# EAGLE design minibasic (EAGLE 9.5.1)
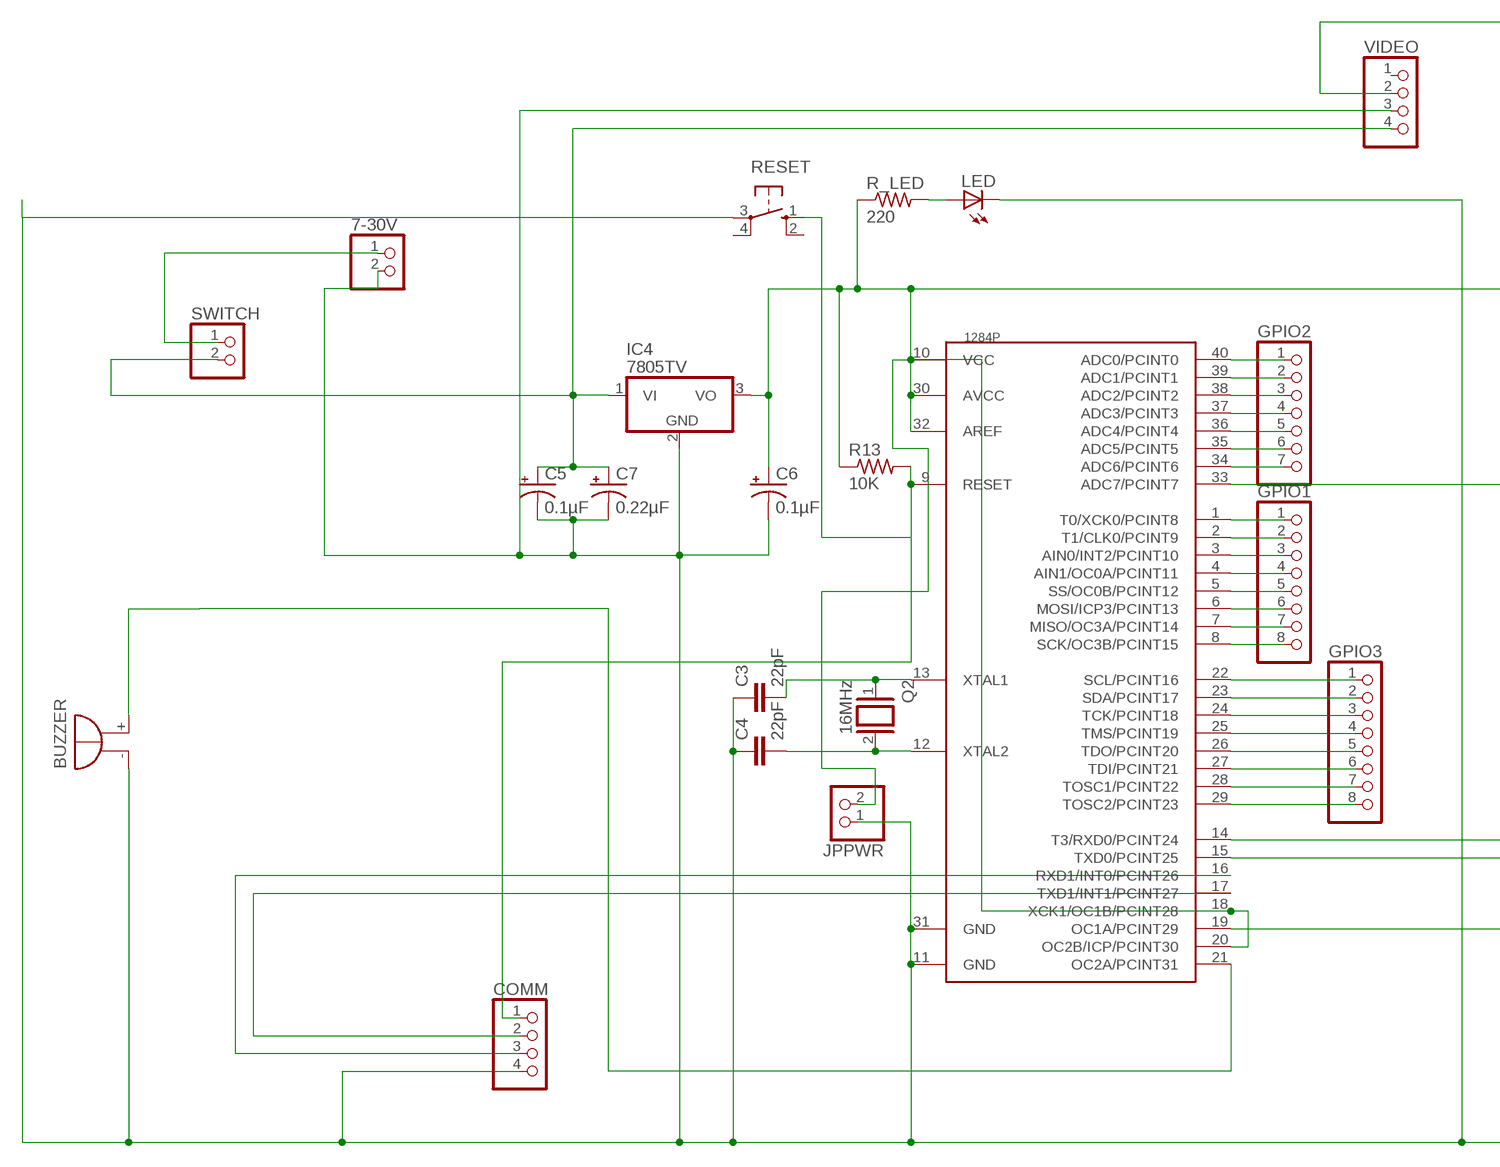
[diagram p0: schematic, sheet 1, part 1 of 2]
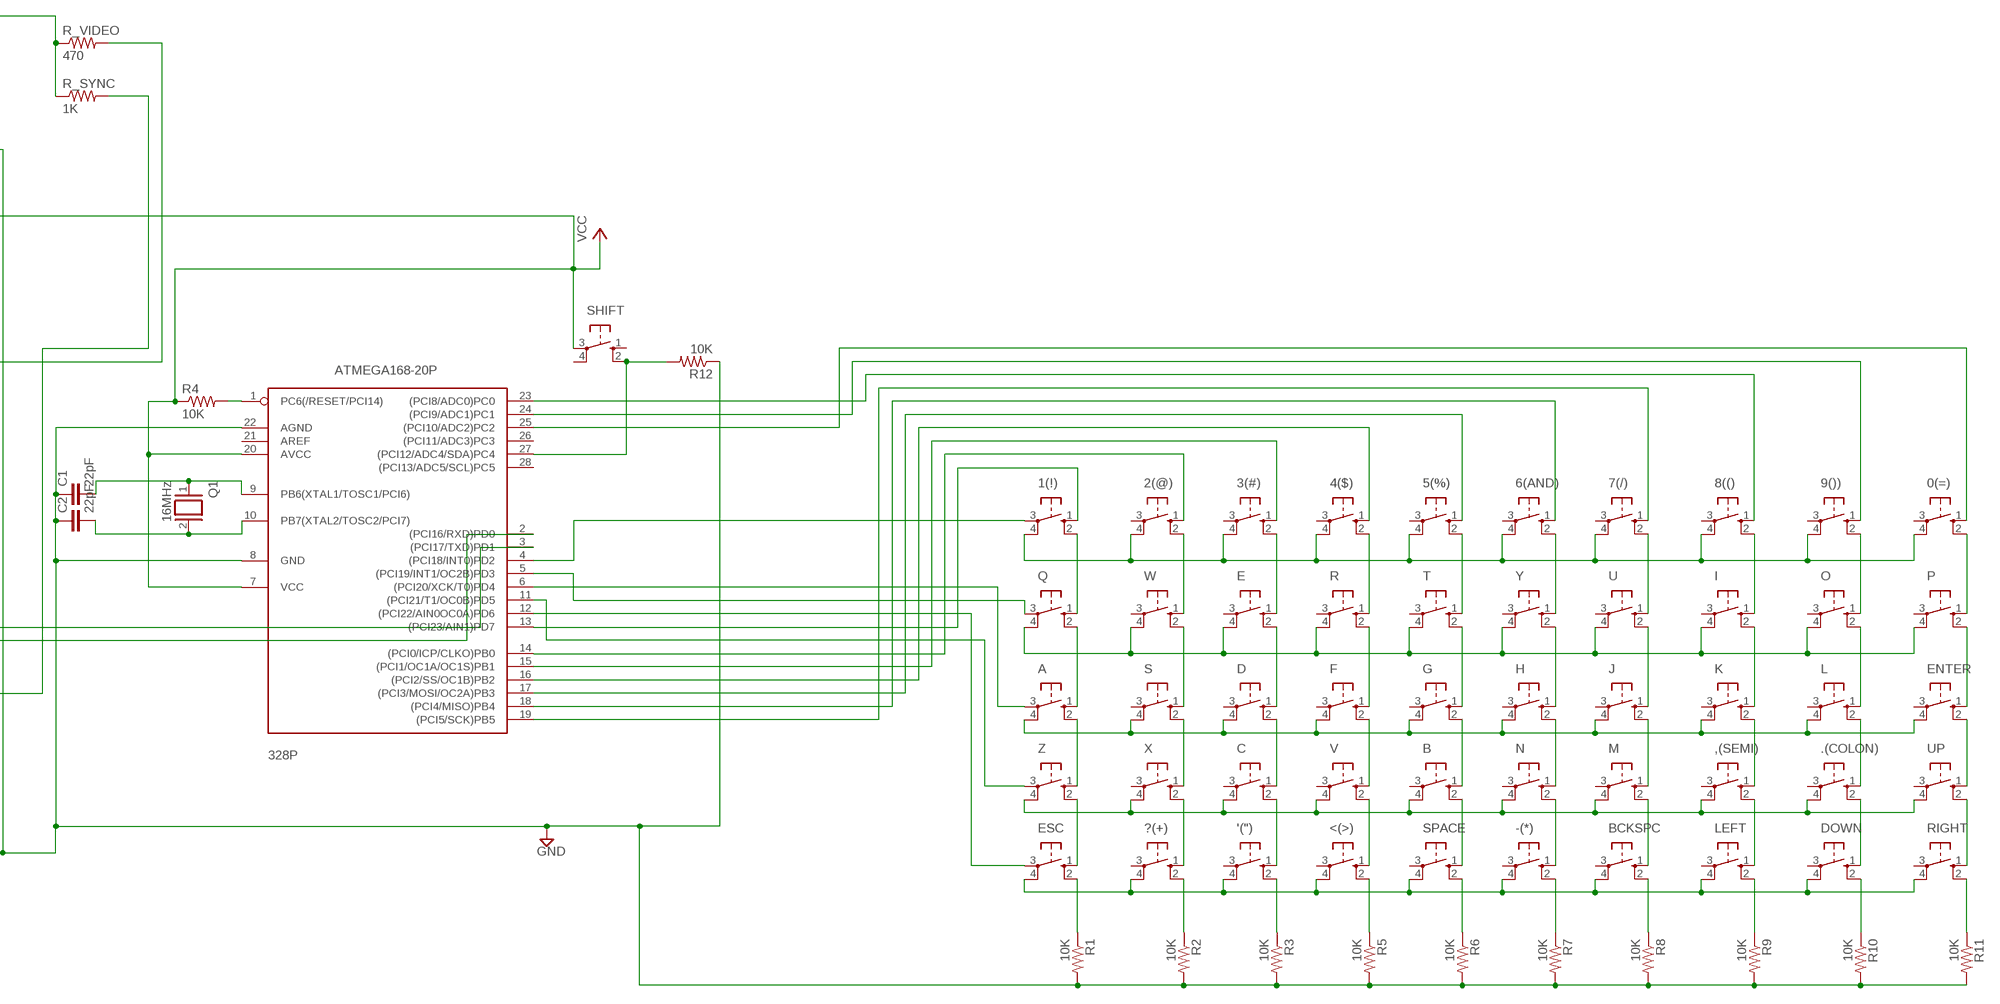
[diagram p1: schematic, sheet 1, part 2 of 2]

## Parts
0(=)  10-XX  [B3F-10XX]
1(!)  10-XX  [B3F-10XX]
2(@)  10-XX  [B3F-10XX]
3(#)  10-XX  [B3F-10XX]
4($)  10-XX  [B3F-10XX]
5(%)  10-XX  [B3F-10XX]
6(AND)  10-XX  [B3F-10XX]
7(/)  10-XX  [B3F-10XX]
7-30V  PINHD-1X2  [1X02]
8(()  10-XX  [B3F-10XX]
9())  10-XX  [B3F-10XX]
328P  ATMEGA168-20P  [DIL28-3]
1284P  MEGA1284P  [DIL40]
'(")  10-XX  [B3F-10XX]
,(SEMI)  10-XX  [B3F-10XX]
-(*)  10-XX  [B3F-10XX]
.(COLON)  10-XX  [B3F-10XX]
<(>)  10-XX  [B3F-10XX]
?(+)  10-XX  [B3F-10XX]
A  10-XX  [B3F-10XX]
B  10-XX  [B3F-10XX]
BCKSPC  10-XX  [B3F-10XX]
BUZZER  F/QMBIII  [F/QMBIII]
C  10-XX  [B3F-10XX]
C1  22pF  C-EU050-050X075  [C050-050X075]
C2  22pF  C-EU050-050X075  [C050-050X075]
C3  22pF  C-EU050-050X075  [C050-050X075]
C4  22pF  C-EU050-050X075  [C050-050X075]
C5  0.1µF  CPOL-USE2-4  [E2-4]
C6  0.1µF  CPOL-USE2-4  [E2-4]
C7  0.22µF  CPOL-USE2.5-5  [E2,5-5]
COMM  PINHD-1X4  [1X04]
D  10-XX  [B3F-10XX]
DOWN  10-XX  [B3F-10XX]
E  10-XX  [B3F-10XX]
ENTER  10-XX  [B3F-10XX]
ESC  10-XX  [B3F-10XX]
F  10-XX  [B3F-10XX]
G  10-XX  [B3F-10XX]
GPIO1  PINHD-1X8  [1X08]
GPIO2  PINHD-1X7  [1X07]
GPIO3  PINHD-1X8  [1X08]
H  10-XX  [B3F-10XX]
I  10-XX  [B3F-10XX]
IC4  7805TV  [TO220V]
J  10-XX  [B3F-10XX]
JPPWR  PINHD-1X2  [1X02]
K  10-XX  [B3F-10XX]
L  10-XX  [B3F-10XX]
LED  LED3MM  [LED3MM]
LEFT  10-XX  [B3F-10XX]
M  10-XX  [B3F-10XX]
N  10-XX  [B3F-10XX]
O  10-XX  [B3F-10XX]
P  10-XX  [B3F-10XX]
Q  10-XX  [B3F-10XX]
Q1  16MHz  XTAL/S  [QS]
Q2  16MHz  XTAL/S  [QS]
R  10-XX  [B3F-10XX]
R1  10K  R-US_0207/10  [0207/10]
R2  10K  R-US_0207/10  [0207/10]
R3  10K  R-US_0207/10  [0207/10]
R4  10K  R-US_0207/10  [0207/10]
R5  10K  R-US_0207/10  [0207/10]
R6  10K  R-US_0207/10  [0207/10]
R7  10K  R-US_0207/10  [0207/10]
R8  10K  R-US_0207/10  [0207/10]
R9  10K  R-US_0207/10  [0207/10]
R10  10K  R-US_0207/10  [0207/10]
R11  10K  R-US_0207/10  [0207/10]
R12  10K  R-US_0207/10  [0207/10]
R13  10K  R-US_0207/10  [0207/10]
R_LED  220  R-US_0207/10  [0207/10]
R_SYNC  1K  R-US_0207/10  [0207/10]
R_VIDEO  470  R-US_0207/10  [0207/10]
RESET  10-XX  [B3F-10XX]
RIGHT  10-XX  [B3F-10XX]
S  10-XX  [B3F-10XX]
SHIFT  10-XX  [B3F-10XX]
SPACE  10-XX  [B3F-10XX]
SWITCH  PINHD-1X2  [1X02]
T  10-XX  [B3F-10XX]
U  10-XX  [B3F-10XX]
UP  10-XX  [B3F-10XX]
V  10-XX  [B3F-10XX]
VIDEO  PINHD-1X4  [1X04]
W  10-XX  [B3F-10XX]
X  10-XX  [B3F-10XX]
Y  10-XX  [B3F-10XX]
Z  10-XX  [B3F-10XX]

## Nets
GND: 7-30V.2 328P.8(GND) 328P.22(AGND) 1284P.11(GND) 1284P.31(GND) BUZZER.-(+) C1.1 C2.1 C3.1 C4.1 C5.- C6.- C7.- COMM.4 IC4.2(GND) JPPWR.1 LED.K(C) R1.2 R2.2 R3.2 R5.2 R6.2 R7.2 R8.2 R9.2 R10.2 R11.2 R12.1 RESET.3(P) VIDEO.3
N$1: 1(!).2(S1) Q.1(S)
N$2: A.1(S) Q.2(S1)
N$3: A.2(S1) Z.1(S)
N$4: ESC.1(S) Z.2(S1)
N$5: 328P.1(PC6(/RESET/PCI14)) R4.2
N$6: ?(+).1(S) X.2(S1)
N$7: S.2(S1) X.1(S)
N$8: 328P.9(PB6(XTAL1/TOSC1/PCI6)) C1.2 Q1.1
N$9: 328P.10(PB7(XTAL2/TOSC2/PCI7)) C2.2 Q1.2
N$10: S.1(S) W.2(S1)
N$11: 2(@).2(S1) W.1(S)
N$12: '(").1(S) C.2(S1)
N$13: C.1(S) D.2(S1)
N$14: D.1(S) E.2(S1)
N$15: 3(#).2(S1) E.1(S)
N$16: 4($).2(S1) R.1(S)
N$17: F.1(S) R.2(S1)
N$18: F.2(S1) V.1(S)
N$19: <(>).1(S) V.2(S1)
N$20: B.2(S1) SPACE.1(S)
N$21: B.1(S) G.2(S1)
N$22: G.1(S) T.2(S1)
N$23: 5(%).2(S1) T.1(S)
N$24: 6(AND).2(S1) Y.1(S)
N$25: H.1(S) Y.2(S1)
N$26: H.2(S1) N.1(S)
N$27: -(*).1(S) N.2(S1)
N$28: BCKSPC.1(S) M.2(S1)
N$29: J.2(S1) M.1(S)
N$30: J.1(S) U.2(S1)
N$31: 7(/).2(S1) U.1(S)
N$32: 8(().2(S1) I.1(S)
N$33: I.2(S1) K.1(S)
N$34: ,(SEMI).1(S) K.2(S1)
N$35: ,(SEMI).2(S1) LEFT.1(S)
N$36: .(COLON).2(S1) DOWN.1(S)
N$37: .(COLON).1(S) L.2(S1)
N$38: L.1(S) O.2(S1)
N$39: 9()).2(S1) O.1(S)
N$40: 0(=).2(S1) P.1(S)
N$41: ENTER.1(S) P.2(S1)
N$42: ENTER.2(S1) UP.1(S)
N$43: RIGHT.1(S) UP.2(S1)
N$44: 0(=).4(P1) 1(!).4(P1) 2(@).4(P1) 3(#).4(P1) 4($).4(P1) 5(%).4(P1) 6(AND).4(P1) 7(/).4(P1) 8(().4(P1) 9()).4(P1)
N$45: 1(!).1(S) 328P.13((PCI23/AIN1)PD7)
N$46: E.4(P1) I.4(P1) O.4(P1) P.4(P1) Q.4(P1) R.4(P1) T.4(P1) U.4(P1) W.4(P1) Y.4(P1)
N$47: A.4(P1) D.4(P1) ENTER.4(P1) F.4(P1) G.4(P1) H.4(P1) J.4(P1) K.4(P1) L.4(P1) S.4(P1)
N$48: ,(SEMI).4(P1) .(COLON).4(P1) B.4(P1) C.4(P1) M.4(P1) N.4(P1) UP.4(P1) V.4(P1) X.4(P1) Z.4(P1)
N$49: '(").4(P1) -(*).4(P1) <(>).4(P1) ?(+).4(P1) BCKSPC.4(P1) DOWN.4(P1) ESC.4(P1) LEFT.4(P1) RIGHT.4(P1) SPACE.4(P1)
N$50: R11.1 RIGHT.2(S1)
N$51: DOWN.2(S1) R10.1
N$52: LEFT.2(S1) R9.1
N$53: BCKSPC.2(S1) R8.1
N$54: -(*).2(S1) R7.1
N$55: R6.1 SPACE.2(S1)
N$56: <(>).2(S1) R5.1
N$57: '(").2(S1) R3.1
N$58: ?(+).2(S1) R2.1
N$59: ESC.2(S1) R1.1
N$60: 2(@).1(S) 328P.14((PCI0/ICP/CLKO)PB0)
N$61: 1(!).3(P) 328P.4((PCI18/INT0)PD2)
N$62: 328P.5((PCI19/INT1/OC2B)PD3) Q.3(P)
N$63: 328P.6((PCI20/XCK/T0)PD4) A.3(P)
N$64: 328P.11((PCI21/T1/OC0B)PD5) Z.3(P)
N$65: 328P.12((PCI22/AIN0OC0A)PD6) ESC.3(P)
N$66: 5(%).1(S) 328P.17((PCI3/MOSI/OC2A)PB3)
N$67: 3(#).1(S) 328P.15((PCI1/OC1A/OC1S)PB1)
N$68: 4($).1(S) 328P.16((PCI2/SS/OC1B)PB2)
N$69: 6(AND).1(S) 328P.18((PCI4/MISO)PB4)
N$70: 7(/).1(S) 328P.19((PCI5/SCK)PB5)
N$71: 8(().1(S) 328P.23((PCI8/ADC0)PC0)
N$72: 9()).1(S) 328P.24((PCI9/ADC1)PC1)
N$73: 0(=).1(S) 328P.25((PCI10/ADC2)PC2)
N$74: 328P.27((PCI12/ADC4/SDA)PC4) R12.2 SHIFT.2(S1)
N$75: R_SYNC.1 R_VIDEO.1 VIDEO.2
N$76: C5.+ C7.+ IC4.1(VI) SWITCH.2 VIDEO.4
N$77: LED.A R_LED.2
N$78: 1284P.12(XTAL2) C4.2 Q2.2
N$79: 1284P.33(ADC7/PCINT7) R_VIDEO.2
N$80: 1284P.13(XTAL1) C3.2 Q2.1
N$81: 1284P.19(OC1A/PCINT29) R_SYNC.2
N$82: 328P.3((PCI17/TXD)PD1) 1284P.14(T3/RXD0/PCINT24)
N$83: 328P.2((PCI16/RXD)PD0) 1284P.15(TXD0/PCINT25)
N$84: 1284P.9(RESET) COMM.1 R13.2 RESET.1(S)
N$85: 7-30V.1 SWITCH.1
N$86: 1284P.16(RXD1/INT0/PCINT26) COMM.3
N$87: 1284P.17(TXD1/INT1/PCINT27) COMM.2
N$88: 1284P.21(OC2A/PCINT31) BUZZER.+(-)
N$89: 1284P.1(T0/XCK0/PCINT8) GPIO1.1
N$90: 1284P.2(T1/CLK0/PCINT9) GPIO1.2
N$91: 1284P.3(AIN0/INT2/PCINT10) GPIO1.3
N$92: 1284P.4(AIN1/OC0A/PCINT11) GPIO1.4
N$93: 1284P.5(SS/OC0B/PCINT12) GPIO1.5
N$94: 1284P.6(MOSI/ICP3/PCINT13) GPIO1.6
N$95: 1284P.7(MISO/OC3A/PCINT14) GPIO1.7
N$96: 1284P.8(SCK/OC3B/PCINT15) GPIO1.8
N$97: 1284P.40(ADC0/PCINT0) GPIO2.1
N$98: 1284P.39(ADC1/PCINT1) GPIO2.2
N$99: 1284P.38(ADC2/PCINT2) GPIO2.3
N$100: 1284P.37(ADC3/PCINT3) GPIO2.4
N$101: 1284P.36(ADC4/PCINT4) GPIO2.5
N$102: 1284P.35(ADC5/PCINT5) GPIO2.6
N$103: 1284P.34(ADC6/PCINT6) GPIO2.7
N$104: 1284P.22(SCL/PCINT16) GPIO3.1
N$105: 1284P.23(SDA/PCINT17) GPIO3.2
N$106: 1284P.24(TCK/PCINT18) GPIO3.3
N$107: 1284P.25(TMS/PCINT19) GPIO3.4
N$108: 1284P.26(TDO/PCINT20) GPIO3.5
N$109: 1284P.27(TDI/PCINT21) GPIO3.6
N$110: 1284P.28(TOSC1/PCINT22) GPIO3.7
N$111: 1284P.29(TOSC2/PCINT23) GPIO3.8
VCC: 328P.7(VCC) 328P.20(AVCC) 1284P.10(VCC) 1284P.18(XCK1/OC1B/PCINT28) 1284P.20(OC2B/ICP/PCINT30) 1284P.30(AVCC) 1284P.32(AREF) C6.+ IC4.3(VO) JPPWR.2 R4.1 R13.1 R_LED.1 SHIFT.3(P)
Unconnected: 0(=).3(P) 2(@).3(P) 3(#).3(P) 4($).3(P) 5(%).3(P) 6(AND).3(P) 7(/).3(P) 8(().3(P) 9()).3(P) 328P.21(AREF) 328P.26((PCI11/ADC3)PC3) 328P.28((PCI13/ADC5/SCL)PC5) '(").3(P) ,(SEMI).3(P) -(*).3(P) .(COLON).3(P) <(>).3(P) ?(+).3(P) B.3(P) BCKSPC.3(P) C.3(P) D.3(P) DOWN.3(P) E.3(P) ENTER.3(P) F.3(P) G.3(P) H.3(P) I.3(P) J.3(P) K.3(P) L.3(P) LEFT.3(P) M.3(P) N.3(P) O.3(P) P.3(P) R.3(P) RESET.2(S1) RESET.4(P1) RIGHT.3(P) S.3(P) SHIFT.1(S) SHIFT.4(P1) SPACE.3(P) T.3(P) U.3(P) UP.3(P) V.3(P) VIDEO.1 W.3(P) X.3(P) Y.3(P)

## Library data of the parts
0(=) 1(!) 2(@) 3(#) 4($) 5(%) 6(AND) 7(/) 8(() 9()) '(") ,(SEMI) -(*) .(COLON) <(>) ?(+) A B BCKSPC C D DOWN E ENTER ESC F G H I J K L LEFT M N O P Q R RESET RIGHT S SHIFT SPACE T U UP V W X Y Z = switch-omron:10-XX: OMRON SWITCH; MPN: B3F-1000; OC_FARNELL: 176432; OC_NEWARK: 36M3542
7-30V JPPWR SWITCH = pinhead:PINHD-1X2: PIN HEADER
328P = adafruit:ATMEGA168*P: MICROCONTROLLER 16 kBytes FLASH 1 kBytes SRAM 512 Bytes EEPROM USART 8-channel 10 bit ADC
1284P = 1284p:MEGA1284P: Atmel ATmega1284P 8-bit AVR Microcontroller
BUZZER = buzzer:F/QMBIII: BUZZER; OC_FARNELL: unknown; OC_NEWARK: unknown
C1-C4 = rcl:C-EU: CAPACITOR, European symbol; SPICEPREFIX: C
C5-C7 = adafruit:CPOL-US: POLARIZED CAPACITOR, American symbol
COMM VIDEO = pinhead:PINHD-1X4: PIN HEADER
GPIO1 GPIO3 = pinhead:PINHD-1X8: PIN HEADER
GPIO2 = pinhead:PINHD-1X7: PIN HEADER
IC4 = linear:78*: Positive VOLTAGE REGULATOR Source: http://cache.national.com/ds/LM/LM78L05.pdf http://www.fairchildsemi.com/ds/LM/LM7805.pdf
LED = adafruit:LED: LED
Q1 Q2 = special:XTAL/S: CRYSTAL
R1-R13 R_LED R_SYNC R_VIDEO = adafruit:R-US_: RESISTOR, American symbol

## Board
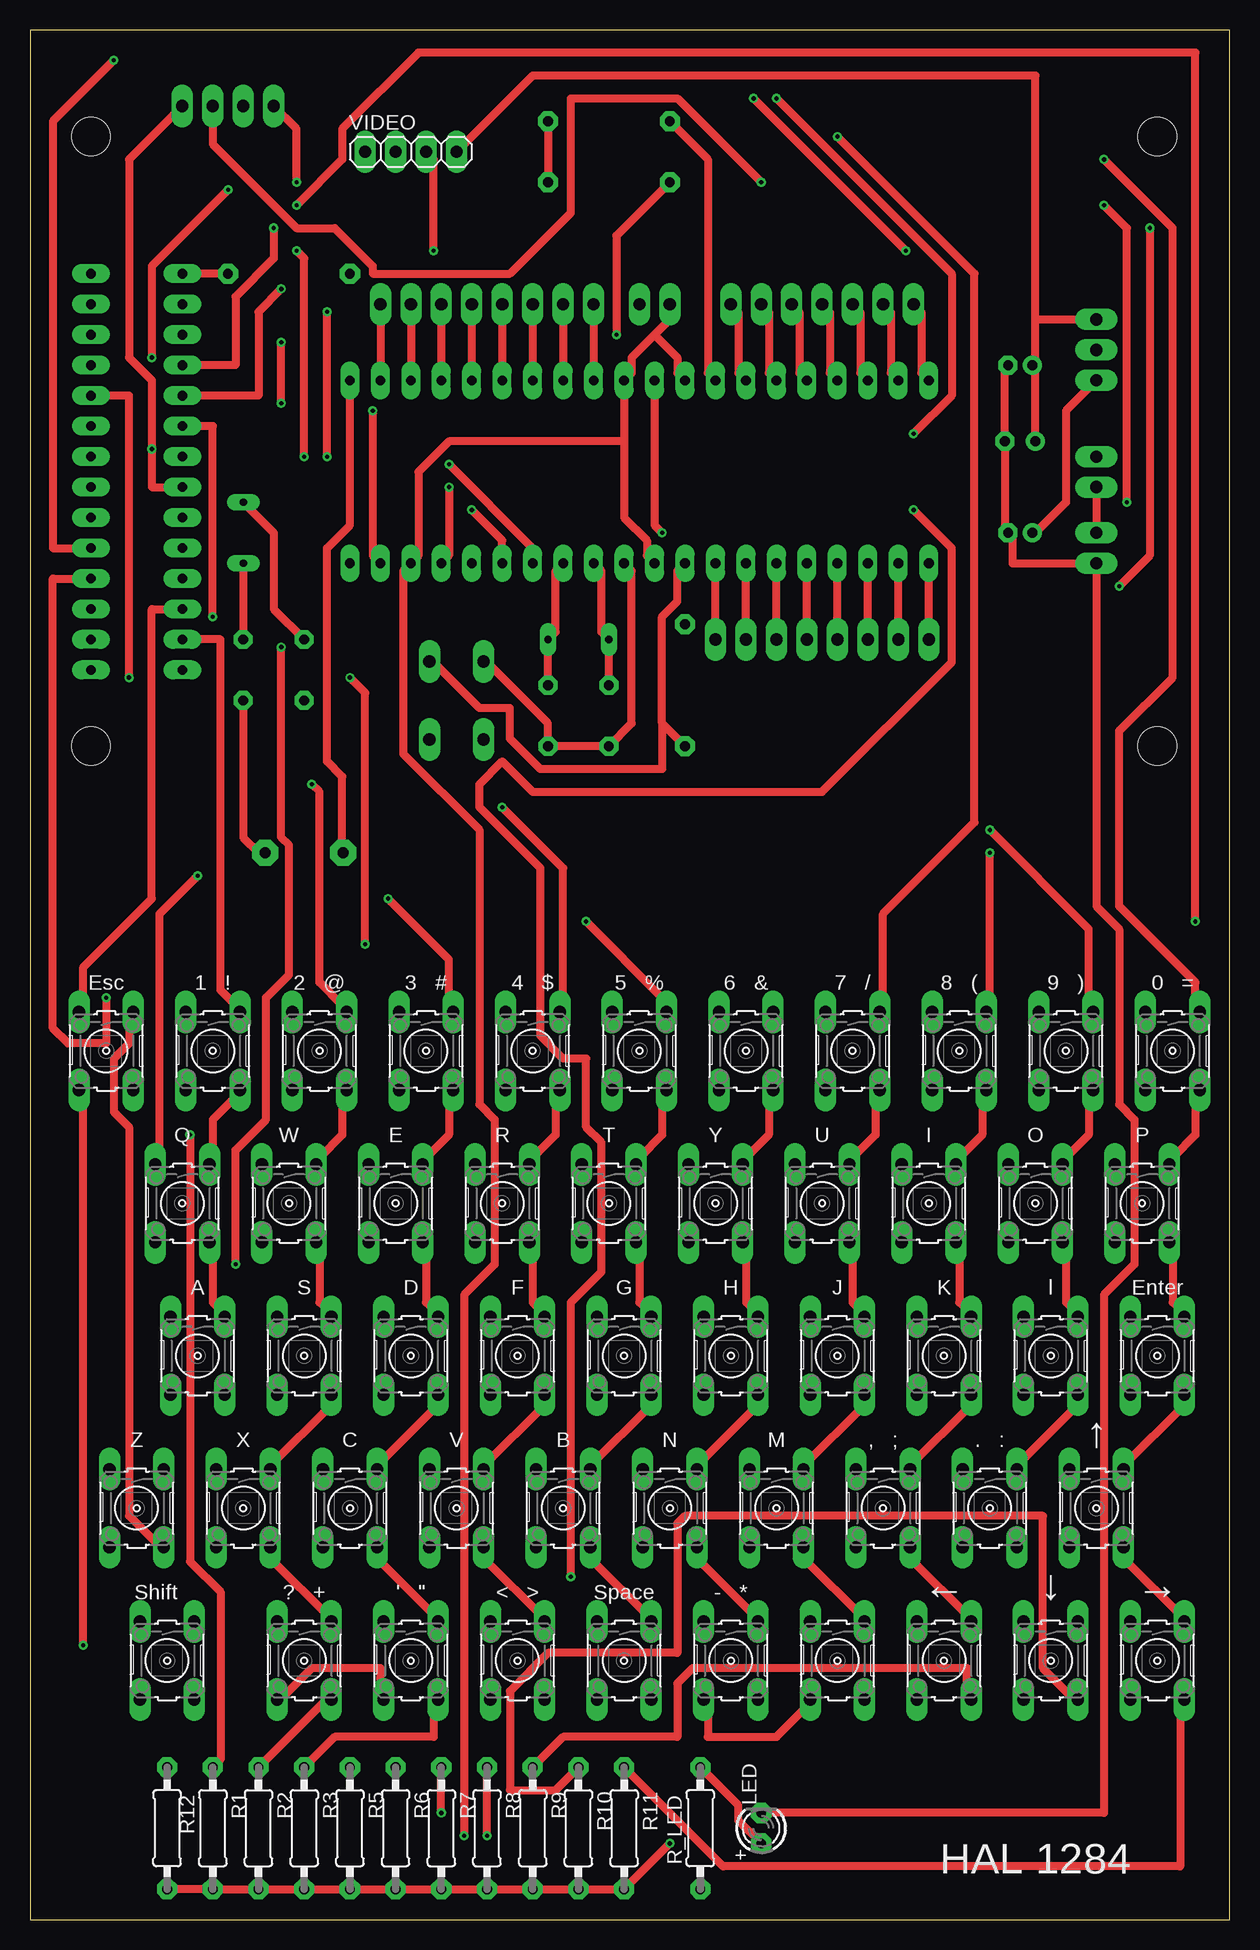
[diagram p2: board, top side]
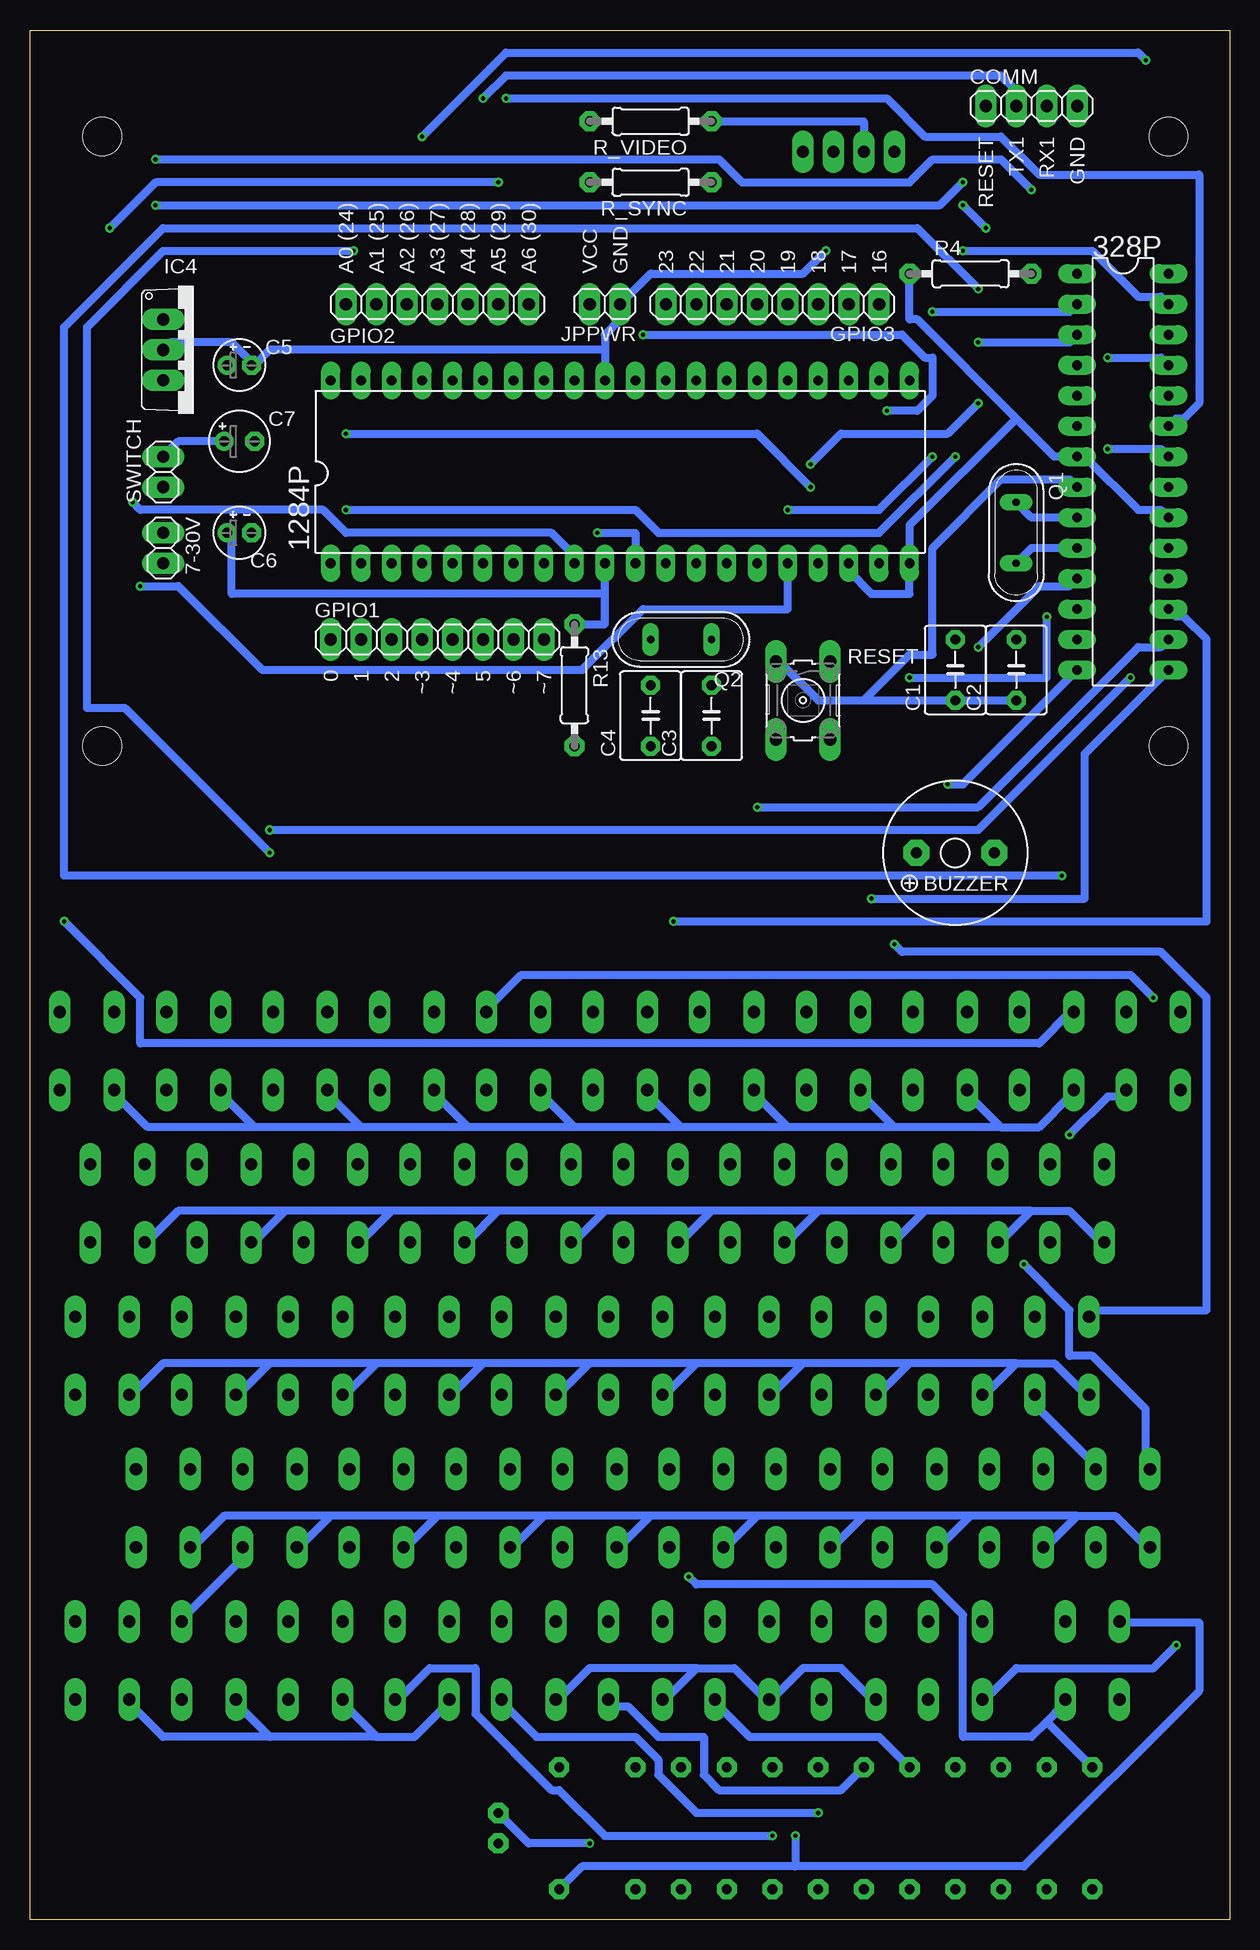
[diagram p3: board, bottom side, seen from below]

Size 100 x 157.47 mm. Coordinates in mm from the lower left corner, seen from the top.
Outline: 0,0 100,0 100,157.47 0,157.47 0,0
Copper layers (1*16): Top 0.035mm / dielectric 1.5mm / Bottom 0.035mm
Design rules "default *": minimum track width 26mil, minimum drill 0.35mm, track to track 26mil, track to pad 16mil, pad to pad 10mil, via to via 6mil, smd to smd 6mil, copper to edge 40mil, drill to drill 6mil, minimum pad ring 15mil, minimum via ring 8mil, stop-mask expansion 4mil, vias tented up to drill 0mil, thermal gap 10mil
Holes 3.2 mm at 5.08,148.59 93.98,148.59 5.08,97.79 93.98,97.79

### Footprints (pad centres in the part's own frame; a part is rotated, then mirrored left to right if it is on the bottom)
B3F-10XX = drill 1.016 long: 1 -3.251,2.261; 2 3.251,2.261; 3 -3.251,-2.261; 4 3.251,-2.261
1X02 = drill 1.016 long: 1 -1.27,0; 2 1.27,0
DIL28-3 = drill 0.813 long: 1 -16.51,-3.81; 2 -13.97,-3.81; 3 -11.43,-3.81; 4 -8.89,-3.81; 5 -6.35,-3.81; 6 -3.81,-3.81; 7 -1.27,-3.81; 8 1.27,-3.81; 9 3.81,-3.81; 10 6.35,-3.81; 11 8.89,-3.81; 12 11.43,-3.81; 13 13.97,-3.81; 14 16.51,-3.81; 15 16.51,3.81; 16 13.97,3.81; 17 11.43,3.81; 18 8.89,3.81; 19 6.35,3.81; 20 3.81,3.81; 21 1.27,3.81; 22 -1.27,3.81; 23 -3.81,3.81; 24 -6.35,3.81; 25 -8.89,3.81; 26 -11.43,3.81; 27 -13.97,3.81; 28 -16.51,3.81
DIL40 = drill 0.813 long: 1 -24.13,-7.62; 2 -21.59,-7.62; 3 -19.05,-7.62; 4 -16.51,-7.62; 5 -13.97,-7.62; 6 -11.43,-7.62; 7 -8.89,-7.62; 8 -6.35,-7.62; 9 -3.81,-7.62; 10 -1.27,-7.62; 11 1.27,-7.62; 12 3.81,-7.62; 13 6.35,-7.62; 14 8.89,-7.62; 15 11.43,-7.62; 16 13.97,-7.62; 17 16.51,-7.62; 18 19.05,-7.62; 19 21.59,-7.62; 20 24.13,-7.62; 21 24.13,7.62; 22 21.59,7.62; 23 19.05,7.62; 24 16.51,7.62; 25 13.97,7.62; 26 11.43,7.62; 27 8.89,7.62; 28 6.35,7.62; 29 3.81,7.62; 30 1.27,7.62; 31 -1.27,7.62; 32 -3.81,7.62; 33 -6.35,7.62; 34 -8.89,7.62; 35 -11.43,7.62; 36 -13.97,7.62; 37 -16.51,7.62; 38 -19.05,7.62; 39 -21.59,7.62; 40 -24.13,7.62
F/QMBIII = drill 0.914 pad 2.159 octagon: + 3.251,0; - -3.251,0
C050-050X075 = drill 0.813 octagon: 1 -2.54,0; 2 2.54,0
E2-4 = drill 0.813 pad 1.422: + -1.016,0 | drill 0.813 pad 1.422 octagon: - 1.016,0
E2,5-5 = drill 0.813 pad 1.6: + -1.27,0 | drill 0.813 pad 1.6 octagon: - 1.27,0
1X04 = drill 1.016 long: 1 -3.81,0; 2 -1.27,0; 3 1.27,0; 4 3.81,0
1X08 = drill 1.016 long: 1 -8.89,0; 2 -6.35,0; 3 -3.81,0; 4 -1.27,0; 5 1.27,0; 6 3.81,0; 7 6.35,0; 8 8.89,0
1X07 = drill 1.016 long: 1 -7.62,0; 2 -5.08,0; 3 -2.54,0; 4 0,0; 5 2.54,0; 6 5.08,0; 7 7.62,0
TO220V = drill 1.016 long: 1 -2.54,-2.54; 2 0,-2.54; 3 2.54,-2.54
LED3MM = drill 0.813 pad 1.676 octagon: A -1.27,0; K 1.27,0
QS = drill 0.61 long: 1 -2.54,0; 2 2.54,0
0207/10 = drill 0.813 pad 1.676 octagon: 1 -5.08,0; 2 5.08,0

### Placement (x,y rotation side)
0(=)  95.25,72.39 270 top
1(!)  15.24,72.39 270 top
2(@)  24.13,72.39 270 top
3(#)  33.02,72.39 270 top
4($)  41.91,72.39 270 top
5(%)  50.8,72.39 270 top
6(AND)  59.69,72.39 270 top
7(/)  68.58,72.39 270 top
7-30V  88.9,114.3 270 bottom
8(()  77.47,72.39 270 top
9())  86.36,72.39 270 top
328P  8.89,120.65 270 bottom
1284P  50.8,120.65 0 bottom
'(")  31.75,21.59 270 top
,(SEMI)  71.12,34.29 270 top
-(*)  58.42,21.59 270 top
.(COLON)  80.01,34.29 270 top
<(>)  40.64,21.59 270 top
?(+)  22.86,21.59 270 top
A  13.97,46.99 270 top
B  44.45,34.29 270 top
BCKSPC  67.31,21.59 270 top
BUZZER  22.86,88.9 180 bottom
C  26.67,34.29 270 top
C1  22.86,104.14 90 bottom
C2  17.78,104.14 90 bottom
C3  43.18,100.33 90 bottom
C4  48.26,100.33 90 bottom
C5  82.55,129.54 0 bottom
C6  82.55,115.57 0 bottom
C7  82.55,123.19 0 bottom
COMM  16.51,151.13 0 bottom
D  31.75,46.99 270 top
DOWN  85.09,21.59 270 top
E  30.48,59.69 270 top
ENTER  93.98,46.99 270 top
ESC  6.35,72.39 270 top
F  40.64,46.99 270 top
G  49.53,46.99 270 top
GPIO1  66.04,106.68 0 bottom
GPIO2  66.04,134.62 0 bottom
GPIO3  38.1,134.62 180 bottom
H  58.42,46.99 270 top
I  74.93,59.69 270 top
IC4  86.36,130.81 270 bottom
J  67.31,46.99 270 top
JPPWR  52.07,134.62 180 bottom
K  76.2,46.99 270 top
L  85.09,46.99 270 top
LED  60.96,7.62 90 top
LEFT  76.2,21.59 270 top
M  62.23,34.29 270 top
N  53.34,34.29 270 top
O  83.82,59.69 270 top
P  92.71,59.69 270 top
Q  12.7,59.69 270 top
Q1  17.78,115.57 270 bottom
Q2  45.72,106.68 180 bottom
R  39.37,59.69 270 top
R1  15.24,7.62 270 top
R2  19.05,7.62 270 top
R3  22.86,7.62 270 top
R4  21.59,137.16 0 bottom
R5  26.67,7.62 270 top
R6  30.48,7.62 270 top
R7  34.29,7.62 270 top
R8  38.1,7.62 270 top
R9  41.91,7.62 270 top
R10  45.72,7.62 270 top
R11  49.53,7.62 270 top
R12  11.43,7.62 90 top
R13  54.61,102.87 270 bottom
R_LED  55.88,7.62 90 top
R_SYNC  48.26,144.78 180 bottom
R_VIDEO  48.26,149.86 180 bottom
RESET  35.56,101.6 270 bottom
RIGHT  93.98,21.59 270 top
S  22.86,46.99 270 top
SHIFT  11.43,21.59 270 top
SPACE  49.53,21.59 270 top
SWITCH  88.9,120.65 90 bottom
T  48.26,59.69 270 top
U  66.04,59.69 270 top
UP  88.9,34.29 270 top
V  35.56,34.29 270 top
VIDEO  31.75,147.32 0 top
W  21.59,59.69 270 top
X  17.78,34.29 270 top
Y  57.15,59.69 270 top
Z  8.89,34.29 270 top

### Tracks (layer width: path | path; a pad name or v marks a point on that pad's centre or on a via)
GND  (via drill 0.35)
  Top 0.66: 328P.8 10.16,119.38 v10.16,122.56 10.16,128.27 8.25,130.18 8.25,146.69 COMM.4 | C2.1 17.78,90.17 19.05,88.9 BUZZER.- | 1284P.11 50.16,112.4 50.16,99.69 C4.1 C3.1 43.18,99.69 38.1,104.78 RESET.3 | R12.1 R1.2 R2.2 R3.2 R5.2 R6.2 R7.2 R8.2 R9.2 R10.2 R11.2 v53.34,6.35 | C5.- 81.28,129.54 C7.- 81.28,115.57 C6.- 81.91,115.57 81.91,113.03 7-30V.2 88.9,84.45 90.8,82.55 90.8,67.94 92.07,66.67 92.07,54.61 89.53,52.07 89.53,8.89 LED.K | VIDEO.3 33.66,146.69 v33.66,139.06 | v52.71,115.57 52.07,116.21 1284P.31
  Bottom 0.66: 328P.22 5.72,122.56 v10.16,122.56 | C2.1 C1.1 30.48,101.6 | 30.48,101.6 34.29,101.6 37.47,104.78 RESET.3 | 328P.8 13.33,120.01 19.05,120.01 24.76,114.3 24.76,105.41 26.67,105.41 30.48,101.6 | LED.K 58.42,6.35 v53.34,6.35 | IC4.2 88.27,131.44 83.19,131.44 81.28,129.54 | 52.07,130.81 52.07,132.08 50.8,133.35 JPPWR.1 48.26,137.16 35.56,137.16 v33.66,139.06 | 52.07,130.81 1284P.31 | 81.28,129.54 80.01,130.81 52.07,130.81 | 81.28,129.54 C5.- | 1284P.11 49.53,115.57 v52.71,115.57
N$1
  Top 0.66: Q.1 15.24,63.5 15.24,66.67 17.14,68.58 1(!).2
N$2
  Top 0.66: A.1 15.88,50.8 15.24,51.44 15.24,55.88 Q.2
N$3
  Bottom 0.66: Z.1 11.43,38.1 16.51,43.18 A.2
N$4
  Top 0.66: Z.2 10.79,31.12 8.25,33.66 8.25,66.04 6.99,67.31 6.99,71.75 8.25,73.03 8.25,75.56 ESC.1
N$5
  Top 0.66: R4.2 328P.1
N$6
  Top 0.66: ?(+).1 24.76,25.4 20.32,29.84 20.32,30.48 X.2
N$7
  Top 0.66: X.1 20.32,38.1 24.76,42.55 24.76,43.18 S.2
N$8
  Top 0.66: C1.2 20.32,109.22 20.32,115.57 Q1.1
  Bottom 0.66: Q1.1 16.51,116.84 328P.9
N$9
  Top 0.66: Q1.2 C2.2
  Bottom 0.66: Q1.2 16.51,114.3 328P.10
N$10
  Top 0.66: S.1 24.76,50.8 24.13,51.44 24.13,55.88 W.2
N$11
  Top 0.66: W.1 24.13,63.5 26.04,65.41 26.04,68.58 2(@).2
N$12
  Top 0.66: '(").1 33.66,25.4 29.21,29.84 29.21,30.48 C.2
N$13
  Top 0.66: C.1 29.21,38.1 33.66,42.55 33.66,43.18 D.2
N$14
  Top 0.66: D.1 33.66,50.8 33.02,51.44 33.02,55.88 E.2
N$15
  Top 0.66: E.1 33.02,63.5 34.93,65.41 34.93,68.58 3(#).2
N$16
  Top 0.66: R.1 41.91,63.5 43.82,65.41 43.82,68.58 4($).2
N$17
  Top 0.66: F.1 42.55,50.8 41.91,51.44 41.91,55.88 R.2
N$18
  Top 0.66: V.1 38.1,38.1 42.55,42.55 42.55,43.18 F.2
N$19
  Top 0.66: <(>).1 42.55,25.4 38.1,29.84 38.1,30.48 V.2
N$20
  Top 0.66: SPACE.1 51.44,25.4 46.99,29.84 46.99,30.48 B.2
N$21
  Top 0.66: B.1 46.99,38.1 51.44,42.55 51.44,43.18 G.2
N$22
  Top 0.66: G.1 51.44,50.8 50.8,51.44 50.8,55.88 T.2
N$23
  Top 0.66: T.1 50.8,63.5 52.71,65.41 52.71,68.58 5(%).2
N$24
  Top 0.66: Y.1 59.69,63.5 61.6,65.41 61.6,68.58 6(AND).2
N$25
  Top 0.66: H.1 60.32,50.8 59.69,51.44 59.69,55.88 Y.2
N$26
  Top 0.66: N.1 55.88,38.1 60.32,42.55 60.32,43.18 H.2
N$27
  Top 0.66: -(*).1 60.32,25.4 55.88,29.84 55.88,30.48 N.2
N$28
  Top 0.66: BCKSPC.1 69.21,25.4 64.77,29.84 64.77,30.48 M.2
N$29
  Top 0.66: M.1 64.77,38.1 69.21,42.55 69.21,43.18 J.2
N$30
  Top 0.66: J.1 69.21,50.8 68.58,51.44 68.58,55.88 U.2
N$31
  Top 0.66: U.1 68.58,63.5 70.48,65.41 70.48,68.58 7(/).2
N$32
  Top 0.66: I.1 77.47,63.5 79.38,65.41 79.38,68.58 8(().2
N$33
  Top 0.66: K.1 78.1,50.8 77.47,51.44 77.47,55.88 I.2
N$34
  Top 0.66: ,(SEMI).1 73.66,38.1 78.1,42.55 78.1,43.18 K.2
N$35
  Top 0.66: LEFT.1 78.1,25.4 73.66,29.84 73.66,30.48 ,(SEMI).2
N$36
  Bottom 0.66: DOWN.1 86.99,25.4 81.91,30.48 .(COLON).2
N$37
  Top 0.66: .(COLON).1 82.55,38.1 86.99,42.55 86.99,43.18 L.2
N$38
  Top 0.66: L.1 86.99,50.8 86.36,51.44 86.36,55.88 O.2
N$39
  Top 0.66: O.1 86.36,63.5 88.27,65.41 88.27,68.58 9()).2
N$40
  Top 0.66: P.1 95.25,63.5 97.16,65.41 97.16,68.58 0(=).2
N$41
  Top 0.66: ENTER.1 95.88,50.8 95.25,51.44 95.25,55.88 P.2
N$42
  Top 0.66: UP.1 91.44,38.1 95.88,42.55 95.88,43.18 ENTER.2
N$43
  Top 0.66: RIGHT.1 95.88,25.4 91.44,29.84 91.44,30.48 UP.2
N$44
  Bottom 0.66: 19.05,66.04 15.88,66.04 13.33,68.58 1(!).4 | 19.05,66.04 21.59,68.58 2(@).4 | 27.94,66.04 30.48,68.58 3(#).4 | 19.05,66.04 27.94,66.04 | 36.83,66.04 39.37,68.58 4($).4 | 27.94,66.04 36.83,66.04 | 45.72,66.04 48.26,68.58 5(%).4 | 36.83,66.04 45.72,66.04 | 54.61,66.04 57.15,68.58 6(AND).4 | 45.72,66.04 54.61,66.04 | 63.5,66.04 66.04,68.58 7(/).4 | 54.61,66.04 63.5,66.04 | 72.39,66.04 74.93,68.58 8(().4 | 63.5,66.04 72.39,66.04 | 81.28,66.04 83.82,68.58 9()).4 | 72.39,66.04 81.28,66.04 | 81.28,66.04 90.17,66.04 92.71,68.58 0(=).4
N$45
  Top 0.66: 328P.13 15.88,106.68 15.88,77.47 17.14,76.2 1(!).1
N$46
  Bottom 0.66: 16.51,59.05 13.33,59.05 10.79,56.52 Q.4 | 16.51,59.05 19.05,56.52 W.4 | 25.4,59.05 27.94,56.52 E.4 | 16.51,59.05 25.4,59.05 | 34.29,59.05 36.83,56.52 R.4 | 25.4,59.05 34.29,59.05 | 43.18,59.05 45.72,56.52 T.4 | 34.29,59.05 43.18,59.05 | 52.07,59.05 54.61,56.52 Y.4 | 43.18,59.05 52.07,59.05 | 60.96,59.05 63.5,56.52 U.4 | 52.07,59.05 60.96,59.05 | 69.85,59.05 72.39,56.52 I.4 | 60.96,59.05 69.85,59.05 | 78.74,59.05 81.28,56.52 O.4 | 69.85,59.05 78.74,59.05 | 78.74,59.05 87.63,59.05 90.17,56.52 P.4
N$47
  Bottom 0.66: 17.78,46.36 14.61,46.36 12.06,43.81 A.4 | 17.78,46.36 20.32,43.81 S.4 | 26.67,46.36 29.21,43.81 D.4 | 17.78,46.36 26.67,46.36 | 35.56,46.36 38.1,43.81 F.4 | 26.67,46.36 35.56,46.36 | 44.45,46.36 46.99,43.81 G.4 | 35.56,46.36 44.45,46.36 | 53.34,46.36 55.88,43.81 H.4 | 44.45,46.36 53.34,46.36 | 62.23,46.36 64.77,43.81 J.4 | 53.34,46.36 62.23,46.36 | 71.12,46.36 73.66,43.81 K.4 | 62.23,46.36 71.12,46.36 | 80.01,46.36 82.55,43.81 L.4 | 71.12,46.36 80.01,46.36 | 80.01,46.36 88.9,46.36 91.44,43.81 ENTER.4
N$48
  Bottom 0.66: 12.7,33.66 9.52,33.66 6.99,31.12 Z.4 | 12.7,33.66 15.24,31.12 X.4 | 21.59,33.66 24.13,31.12 C.4 | 12.7,33.66 21.59,33.66 | 30.48,33.66 33.02,31.12 V.4 | 21.59,33.66 30.48,33.66 | 39.37,33.66 41.91,31.12 B.4 | 30.48,33.66 39.37,33.66 | 48.26,33.66 50.8,31.12 N.4 | 39.37,33.66 48.26,33.66 | 57.15,33.66 59.69,31.12 M.4 | 48.26,33.66 57.15,33.66 | 66.04,33.66 68.58,31.12 ,(SEMI).4 | 57.15,33.66 66.04,33.66 | 74.93,33.66 77.47,31.12 .(COLON).4 | 66.04,33.66 74.93,33.66 | 74.93,33.66 83.82,33.66 86.36,31.12 UP.4
N$49  (via drill 0.35)
  Top 0.66: ?(+).4 20.95,18.41 23.49,20.95 29.21,20.95 29.21,18.41 '(").4 | v4.44,22.86 4.44,68.58 ESC.4 | BCKSPC.4 64.77,17.78 62.23,15.24 56.52,15.24 56.52,17.78 -(*).4
  Bottom 0.66: 71.12,15.24 67.94,15.24 65.41,17.78 BCKSPC.4 | 71.12,15.24 73.66,17.78 LEFT.4 | 80.01,15.24 82.55,17.78 DOWN.4 | 71.12,15.24 80.01,15.24 | 80.01,15.24 88.9,15.24 91.44,17.78 RIGHT.4 | 44.45,20.95 41.28,20.95 38.73,18.41 <(>).4 38.1,18.41 35.56,20.95 32.39,20.95 29.85,18.41 '(").4 | 44.45,20.95 46.99,18.41 SPACE.4 | 44.45,20.95 53.34,20.95 55.88,18.41 -(*).4 | v4.44,22.86 6.35,20.95 17.78,20.95 20.32,18.41 ?(+).4
N$50
  Top 0.66: R11.1 57.79,4.45 95.88,4.45 95.88,17.78 RIGHT.2
N$51
  Top 0.66: R10.1 43.82,10.79 40.01,10.79 40.01,19.05 43.18,22.23 53.98,22.23 53.98,33.02 54.61,33.66 84.45,33.66 84.45,20.95 86.99,18.41 DOWN.2
N$52
  Top 0.66: R9.1 44.45,15.24 53.98,15.24 53.98,19.69 55.25,20.95 78.1,20.95 78.1,18.41 LEFT.2
N$53  (via drill 0.35)
  Top 0.66: v38.1,6.98 R8.1
  Bottom 0.66: v38.1,6.98 52.07,6.98 55.88,10.79 56.52,10.79 62.87,17.14 62.87,20.95 66.67,20.95 69.21,18.41 BCKSPC.2
N$54  (via drill 0.35)
  Top 0.66: v34.29,8.89 R7.1
  Bottom 0.66: v34.29,8.89 44.45,8.89 47.62,12.06 47.62,13.33 49.53,15.24 57.79,15.24 60.32,17.78 -(*).2
N$55
  Bottom 0.66: R6.1 32.39,10.79 42.55,10.79 43.82,12.06 43.82,15.24 47.62,15.24 50.16,17.78 51.44,17.78 SPACE.2
N$56
  Bottom 0.66: R5.1 29.21,15.24 40.01,15.24 42.55,17.78 <(>).2
N$57
  Top 0.66: R3.1 25.4,15.24 33.66,15.24 33.66,17.78 '(").2
N$58
  Top 0.66: R2.1 24.76,18.41 ?(+).2
N$59  (via drill 0.35)
  Top 0.66: R1.1 15.88,13.33 15.88,27.3 13.33,29.84 v13.33,65.41
  Bottom 0.66: v13.33,65.41 10.16,68.58 8.89,68.58 ESC.2
N$60  (via drill 0.35)
  Top 0.66: v23.49,94.61 24.13,93.98 24.13,78.11 26.04,76.2 2(@).1
  Bottom 0.66: 328P.14 22.22,94.61 v23.49,94.61
N$61  (via drill 0.35)
  Top 0.66: 328P.4 17.14,129.54 17.14,135.25 20.32,138.43 v20.32,140.97 | v22.22,142.88 26.04,146.69 26.04,149.22 32.39,155.57 97.16,155.57 v97.16,83.19
  Bottom 0.66: v22.22,142.88 v20.32,140.97 | v97.16,83.19 90.8,76.83 90.8,73.03 15.88,73.03 13.33,75.56 1(!).3
N$62  (via drill 0.35)
  Top 0.66: 328P.5 19.05,127 19.05,133.98 v20.95,135.89 | v13.97,87 10.79,83.82 10.79,63.5 Q.3
  Bottom 0.66: v20.95,135.89 26.04,140.97 88.9,140.97 97.16,132.72 97.16,87 v13.97,87
N$63  (via drill 0.35)
  Top 0.66: 328P.6 15.24,124.46 v15.24,108.58 | v26.67,103.5 27.94,102.23 v27.94,81.28
  Bottom 0.66: v15.24,108.58 15.24,103.5 v26.67,103.5 | v27.94,81.28 27.3,80.64 5.72,80.64 1.91,76.83 1.91,50.8 11.43,50.8 A.3
N$64  (via drill 0.35)
  Top 0.66: v20.95,106.05 20.95,90.17 21.59,89.53 21.59,78.74 19.68,76.83 19.68,66.67 17.14,64.14 v17.14,54.61
  Bottom 0.66: 328P.11 13.33,111.12 15.88,111.12 v20.95,106.05 | v17.14,54.61 13.33,50.8 13.33,46.99 11.43,46.99 6.99,42.55 6.99,38.1 Z.3
N$65
  Top 0.66: 328P.12 10.16,109.22 10.16,85.09 4.44,79.38 4.44,76.2 ESC.3
N$66  (via drill 0.35)
  Top 0.66: v46.36,83.19 52.71,76.83 52.71,76.2 5(%).1
  Bottom 0.66: 328P.17 4.44,108.58 3.81,108.58 1.91,106.68 1.91,83.19 v46.36,83.19
N$67  (via drill 0.35)
  Top 0.66: v29.85,85.09 34.93,80.01 34.93,76.2 3(#).1
  Bottom 0.66: 328P.15 12.06,97.16 12.06,85.09 v29.85,85.09
N$68  (via drill 0.35)
  Top 0.66: v39.37,92.71 44.45,87.63 44.45,76.2 4($).1
  Bottom 0.66: 328P.16 5.72,106.05 7.62,106.05 20.95,92.71 v39.37,92.71
N$69  (via drill 0.35)
  Top 0.66: 328P.18 1.91,111.76 1.91,74.3 3.17,73.03 6.35,73.03 v6.35,76.83
  Bottom 0.66: v6.35,76.83 8.25,78.74 59.05,78.74 61.6,76.2 6(AND).1
N$70  (via drill 0.35)
  Top 0.66: 328P.19 1.91,114.3 1.91,149.86 v6.99,154.94 | v67.31,148.59 78.74,137.16 78.74,91.44 71.12,83.82 71.12,76.2 7(/).1
  Bottom 0.66: v6.99,154.94 7.62,155.57 60.32,155.57 v67.31,148.59
N$71  (via drill 0.35)
  Top 0.66: v73.02,139.06 v60.32,151.76 | v80.01,88.9 80.01,76.2 8(().1
  Bottom 0.66: 328P.23 4.44,125.09 3.81,125.09 2.54,126.37 2.54,145.41 15.88,145.41 19.05,148.59 25.4,148.59 28.57,151.76 v60.32,151.76 | v73.02,139.06 88.9,139.06 95.25,132.72 95.25,100.97 92.07,100.97 v80.01,88.9
N$72  (via drill 0.35)
  Top 0.66: 328P.24 8.25,127 v8.25,103.5 | v80.01,90.8 88.27,82.55 88.27,76.2 9()).1
  Bottom 0.66: v8.25,103.5 20.95,90.8 v80.01,90.8
N$73  (via drill 0.35)
  Top 0.66: v10.16,130.18 10.16,137.79 v16.51,144.15 | v89.53,146.69 95.25,140.97 95.25,103.5 90.8,99.06 90.8,84.45 97.16,78.11 97.16,76.2 0(=).1
  Bottom 0.66: 328P.25 5.72,130.18 v10.16,130.18 | v16.51,144.15 19.05,146.69 24.76,146.69 26.67,144.78 40.64,144.78 42.55,146.69 v89.53,146.69
N$74  (via drill 0.35)
  Top 0.66: v22.22,139.06 22.86,138.43 v22.86,121.92 | v73.66,117.47 76.83,114.3 76.83,104.78 66.04,93.98 41.91,93.98 39.37,96.52 37.47,94.61 37.47,92.71 42.55,87.63 42.55,73.66 44.45,71.75 46.36,71.75 46.36,66.04 47.62,64.77 47.62,53.97 45.09,51.44 v45.09,28.57
  Bottom 0.66: 328P.27 5.72,135.25 7.62,135.25 11.43,139.06 v22.22,139.06 | v22.86,121.92 29.21,115.57 47.62,115.57 49.53,117.47 v73.66,117.47 | v45.09,28.57 44.45,27.94 24.76,27.94 22.22,25.4 22.22,15.24 16.51,15.24 15.24,16.51 | 15.24,16.51 13.97,17.78 SHIFT.2 | 15.24,16.51 R12.2
N$75
  Top 0.66: R_VIDEO.1 R_SYNC.1
  Bottom 0.66: VIDEO.2 30.48,149.86 R_VIDEO.1
N$76
  Top 0.66: C7.+ 83.82,129.54 | 83.82,133.35 IC4.1 | 83.82,129.54 83.82,133.35 | 83.82,129.54 C5.+ | VIDEO.4 41.91,153.67 83.82,153.67 83.82,133.35
  Bottom 0.66: SWITCH.2 87.63,123.19 C7.+
N$77
  Top 0.66: R_LED.2 59.05,9.52 59.05,8.25 LED.A
N$78
  Top 0.66: C4.2 Q2.2 47.62,107.31 47.62,112.4 1284P.12
N$79
  Top 0.66: 1284P.33 56.52,128.91 56.52,146.69 R_VIDEO.2
N$80
  Top 0.66: C3.2 Q2.1 43.82,107.31 43.82,112.4 1284P.13
N$81  (via drill 0.35)
  Top 0.66: 1284P.19 28.57,113.66 v28.57,125.73 | v48.9,132.08 48.9,140.34 R_SYNC.2
  Bottom 0.66: v28.57,125.73 26.04,125.73 24.76,127 24.76,130.18 25.4,130.18 27.3,132.08 v48.9,132.08
N$82  (via drill 0.35)
  Top 0.66: v20.95,126.37 v20.95,131.44 | v34.93,121.28 41.91,114.3 1284P.14
  Bottom 0.66: 328P.3 13.33,131.44 v20.95,131.44 | v20.95,126.37 23.49,123.82 32.39,123.82 v34.93,121.28
N$83  (via drill 0.35)
  Top 0.66: v24.76,121.92 v24.76,133.98 | v36.83,117.47 39.37,114.94 1284P.15
  Bottom 0.66: 328P.2 13.33,133.98 v24.76,133.98 | v24.76,121.92 29.21,117.47 v36.83,117.47
N$84  (via drill 0.35)
  Top 0.66: 1284P.9 53.98,112.4 53.98,109.86 52.71,108.58 52.71,99.69 | R13.2 52.71,99.69 | 52.71,99.69 52.71,95.89 42.55,95.89 40.01,98.42 40.01,100.97 37.47,100.97 33.66,104.78 RESET.1 | COMM.1 22.22,149.22 v22.22,144.78 | v89.53,142.88 91.44,140.97 v91.44,118.11
  Bottom 0.66: v22.22,144.78 24.13,142.88 v89.53,142.88 | v91.44,118.11 90.8,117.47 75.56,117.47 73.66,115.57 56.52,115.57 54.61,113.66 1284P.9
N$85
  Top 0.66: SWITCH.1 7-30V.1
N$86  (via drill 0.35)
  Top 0.66: v90.8,111.12 93.34,113.66 v93.34,140.97 | v60.96,144.78 53.98,151.76 45.09,151.76 45.09,142.24 40.01,137.16 28.57,137.16 28.57,137.79 25.4,140.97 22.22,140.97 15.24,147.96 COMM.3
  Bottom 0.66: 1284P.16 36.83,109.22 48.9,109.22 53.98,104.14 80.64,104.14 87.63,111.12 v90.8,111.12 | v93.34,140.97 89.53,144.78 v60.96,144.78
N$87  (via drill 0.35)
  Top 0.66: 1284P.17 34.93,113.66 v34.93,119.38 | v73.66,123.82 76.83,127 76.83,137.16 v62.23,151.76
  Bottom 0.66: v34.93,119.38 39.37,123.82 v73.66,123.82 | v62.23,151.76 60.32,153.67 19.05,153.67 17.78,152.4 COMM.2
N$88
  Top 0.66: 1284P.21 26.67,116.21 24.76,114.3 24.76,96.52 26.04,95.25 26.04,88.9 BUZZER.+
N$89
  Top 0.66: GPIO1.1 1284P.1
N$90
  Top 0.66: GPIO1.2 1284P.2
N$91
  Top 0.66: GPIO1.3 1284P.3
N$92
  Top 0.66: GPIO1.4 1284P.4
N$93
  Top 0.66: GPIO1.5 1284P.5
N$94
  Top 0.66: GPIO1.6 1284P.6
N$95
  Top 0.66: GPIO1.7 1284P.7
N$96
  Top 0.66: GPIO1.8 1284P.8
N$97
  Top 0.66: 1284P.40 74.3,128.91 74.3,133.98 GPIO2.1
N$98
  Top 0.66: 1284P.39 71.75,128.91 71.75,133.98 GPIO2.2
N$99
  Top 0.66: 1284P.38 69.21,128.91 69.21,133.98 GPIO2.3
N$100
  Top 0.66: 1284P.37 66.67,128.91 66.67,133.98 GPIO2.4
N$101
  Top 0.66: 1284P.36 64.13,128.91 64.13,133.98 GPIO2.5
N$102
  Top 0.66: 1284P.35 61.6,128.91 61.6,133.98 GPIO2.6
N$103
  Top 0.66: 1284P.34 59.05,128.91 59.05,133.98 GPIO2.7
N$104
  Top 0.66: GPIO3.1 1284P.22
N$105
  Top 0.66: GPIO3.2 1284P.23
N$106
  Top 0.66: GPIO3.3 1284P.24
N$107
  Top 0.66: GPIO3.4 1284P.25
N$108
  Top 0.66: GPIO3.5 1284P.26
N$109
  Top 0.66: GPIO3.6 1284P.27
N$110
  Top 0.66: GPIO3.7 1284P.28
N$111
  Top 0.66: GPIO3.8 1284P.29
VCC  (via drill 0.35)
  Top 0.66: IC4.3 86.36,125.73 86.36,118.11 83.82,115.57 C6.+ | 52.07,132.08 53.34,133.35 JPPWR.2 | 52.07,132.08 50.16,130.18 50.16,128.91 1284P.30 49.53,123.19 | 1284P.32 53.98,128.91 53.98,130.18 52.07,132.08 | 1284P.10 51.44,113.66 51.44,114.94 49.53,116.84 49.53,123.19 | 49.53,123.19 34.93,123.19 32.39,120.65 32.39,113.66 1284P.18 31.11,112.4 31.11,97.16 37.47,90.8 37.47,67.94 38.73,66.67 38.73,54.61 36.2,52.07 v36.2,6.98
  Bottom 0.66: R_LED.1 53.98,4.45 36.2,4.45 | 36.2,4.45 17.14,4.45 2.54,19.05 2.54,24.77 8.89,24.77 SHIFT.3 | 1284P.18 31.75,112.4 29.85,110.49 26.67,110.49 1284P.20 26.67,116.21 17.78,125.09 | 328P.20 5.72,117.47 7.62,117.47 12.06,121.92 328P.7 14.61,121.92 17.78,125.09 | R4.1 26.67,133.35 26.04,133.35 17.78,125.09 | 52.07,110.49 52.07,107.95 R13.1 | 52.07,110.49 1284P.10 | 52.07,110.49 83.19,110.49 83.19,115.57 C6.+ | v36.2,6.98 36.2,4.45

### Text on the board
tNames: Esc | 1 ! | 2 @ | 3 # | 4 $ | 5 % | 6 & | 7 / | 8 ( | 9 ) | 0 = | Q | W | E | R | T | Y | U | I | O | P | A | S | D | F | G | H | J | K | l | Enter | Z | X | C | V | B | N | M | , ; | . : | ↑ | Shift ⇑ | ? + | ' " | < > | Space | - * | ⇤ | ← | ↓ | → | HAL 1284
bNames: GND | RX1 | TX1 | RESET | 16 | 17 | 18 | 19 | 20 | 21 | 22 | 23 | GND | VCC | A6 (30) | A5 (29) | A4 (28) | A3 (27) | A2 (26) | A1 (25) | A0 (24) | ~7 | ~6 | 5 | ~4 | ~3 | 2 | 1 | 0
